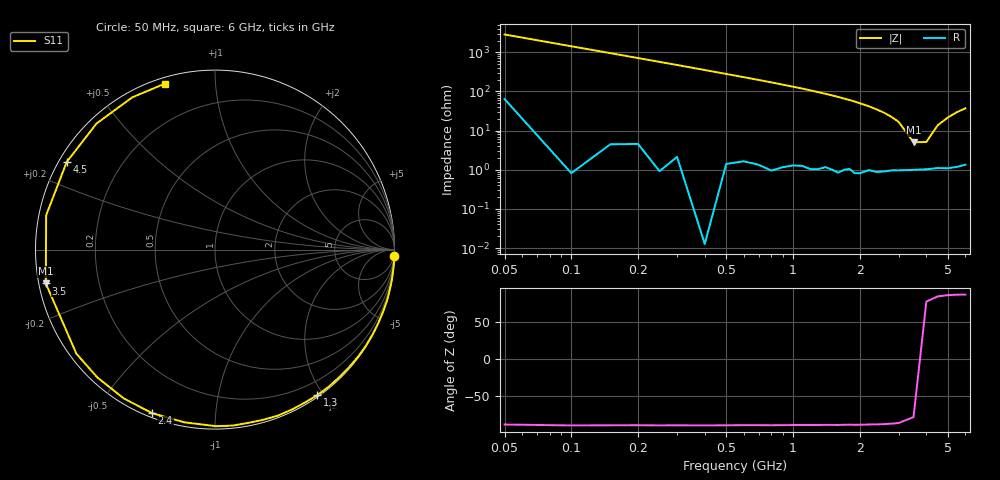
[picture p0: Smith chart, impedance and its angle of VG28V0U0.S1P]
! Infineon Technologies  Discrete & RF Semiconductors
! BB 831
! Si Tuning Diode in SOD323
! VR = 28 V
! S-Parameters:  July  1999
# GHz  S  MA  R  50
!  f  S11
! GHz  MAG  ANG
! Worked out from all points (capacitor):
!   34 points, 50 MHz to 6 GHz, reference 50 ohm
!   read as one part to ground: C = 1.11 pF near 50 MHz
!   lowest |Z| = 5.04 ohm at 3.5 GHz (marker M1)
!   series resonance near 3.748 GHz, so ESL is about 1.6 nH
!   S11 on the Smith chart (normalised r, x): 50 MHz: 1, -57; 1.3 GHz: 0.02, -1.92; 2.4 GHz: 0.02, -0.69; 3.5 GHz: 0.02, -0.10; 4.5 GHz: 0.02, +0.27; 6 GHz: 0.03, +0.74
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0.05  0.9992 -2.0
0.15  0.9995 -6.0
0.25  0.9997 -10.0
0.4  1 -16.1
0.6  0.9971 -24.3
0.7  0.9968 -28.4
0.8  0.997 -32.7
0.9  0.9953 -37.0
1.1  0.9925 -45.6
1.2  0.9926 -50.2
1.3  0.9912 -54.9
1.5  0.9887 -64.2
1.6  0.9892 -69.2
1.7  0.9856 -74.3
1.8  0.9831 -79.1
1.9  0.9853 -84.2
2  0.984 -89.6
2.2  0.9774 -100.0
2.4  0.9764 -111.0
2.6  0.9726 -121.5
2.8  0.968 -132.6
3  0.9658 -143.1
3.5  0.9613 -168.7
4  0.96 168.5
4.5  0.9596 149.4
5  0.9639 133.2
5.5  0.9654 118.5
6  0.9658 106.8
